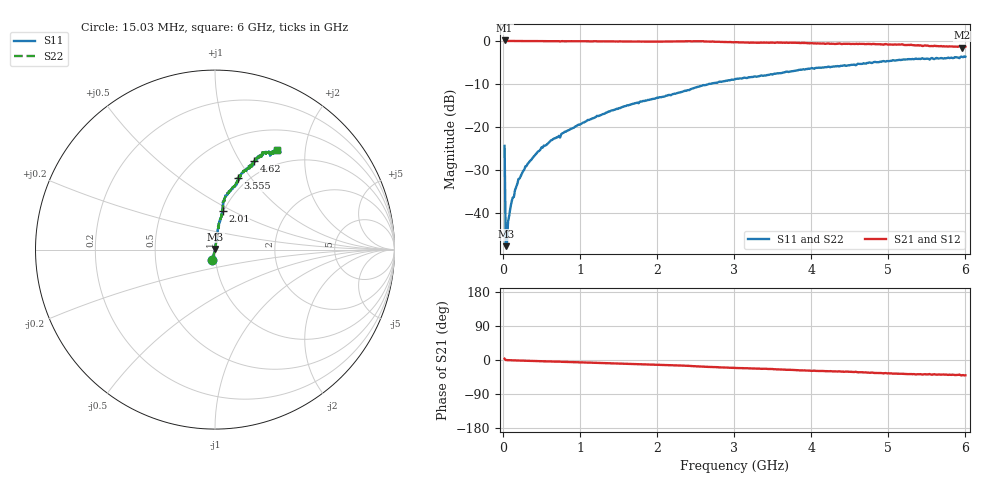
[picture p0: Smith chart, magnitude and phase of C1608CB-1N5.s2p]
!	Network	Analyzer	HP8753E.07.74:	Oct	30	2002	Serial	No.	JP38451487
!	Hewlett-Packard
!	7	Sep	2009	9:29:01
!	Frequency	S11	S21	S12	S22
#	HZ	S	RI	R	50
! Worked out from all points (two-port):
!   400 points, 15.03 MHz to 6 GHz, reference 50 ohm
!   highest |S21| = 0.10 dB at 15.03 MHz (marker M1); lowest = -1.6 dB at 5.955 GHz (marker M2)
!   |S21| within 3 dB of the highest: start of sweep to end of sweep
!   lowest |S11| = -47.8 dB at 30.03 MHz (marker M3), VSWR 1.01, Z = 50.1 + j0.393 ohm
!   |S11| at or under -10 dB: start of sweep to 2.67 GHz
!   |S22| runs from -47.8 to -3.6 dB; largest |S21 - S12| = 0
!   S11 on the Smith chart (normalised r, x): 15.03 MHz: 0.96, -0.11; 2.01 GHz: 0.99, +0.44; 3.555 GHz: 0.89, +0.87; 4.62 GHz: 0.83, +1.15; 6 GHz: 0.78, +1.51
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1.502992e7  -0.0145 -0.0583  1.01 0.0583  1.01 0.0583  -0.0145 -0.0583
3.002985e7  0.00119 0.00392  0.999 -0.00392  0.999 -0.00392  0.00119 0.00392
4.502978e7  0.000675 0.00416  0.999 -0.00416  0.999 -0.00416  0.000675 0.00416
6.00297e7  0.00166 0.00777  0.998 -0.00777  0.998 -0.00777  0.00166 0.00777
1.050295e8  0.00262 0.0131  0.997 -0.0131  0.997 -0.0131  0.00262 0.0131
1.350293e8  0.00348 0.0149  0.997 -0.0149  0.997 -0.0149  0.00348 0.0149
1.500292e8  0.003 0.0181  0.997 -0.0181  0.997 -0.0181  0.003 0.0181
1.95029e8  0.00301 0.0245  0.997 -0.0245  0.997 -0.0245  0.00301 0.0245
2.850286e8  0.005 0.0344  0.995 -0.0344  0.995 -0.0344  0.005 0.0344
4.950275e8  0.00624 0.0576  0.994 -0.0576  0.994 -0.0576  0.00624 0.0576
1.020025e9  0.0155 0.109  0.985 -0.109  0.985 -0.109  0.0155 0.109
1.410023e9  0.024 0.154  0.976 -0.154  0.976 -0.154  0.024 0.154
2.01002e9  0.0427 0.214  0.957 -0.214  0.957 -0.214  0.0427 0.214
3.015015e9  0.0983 0.347  0.902 -0.347  0.902 -0.347  0.0983 0.347
3.555012e9  0.127 0.4  0.873 -0.4  0.873 -0.4  0.127 0.4
4.00501e9  0.175 0.451  0.825 -0.451  0.825 -0.451  0.175 0.451
4.620007e9  0.218 0.494  0.782 -0.494  0.782 -0.494  0.218 0.494
5.010005e9  0.256 0.522  0.744 -0.522  0.744 -0.522  0.256 0.522
5.445003e9  0.318 0.541  0.682 -0.541  0.682 -0.541  0.318 0.541
5.925e9  0.318 0.544  0.682 -0.544  0.682 -0.544  0.318 0.544
5.955e9  0.364 0.543  0.636 -0.543  0.636 -0.543  0.364 0.543
6e9  0.348 0.554  0.652 -0.554  0.652 -0.554  0.348 0.554
